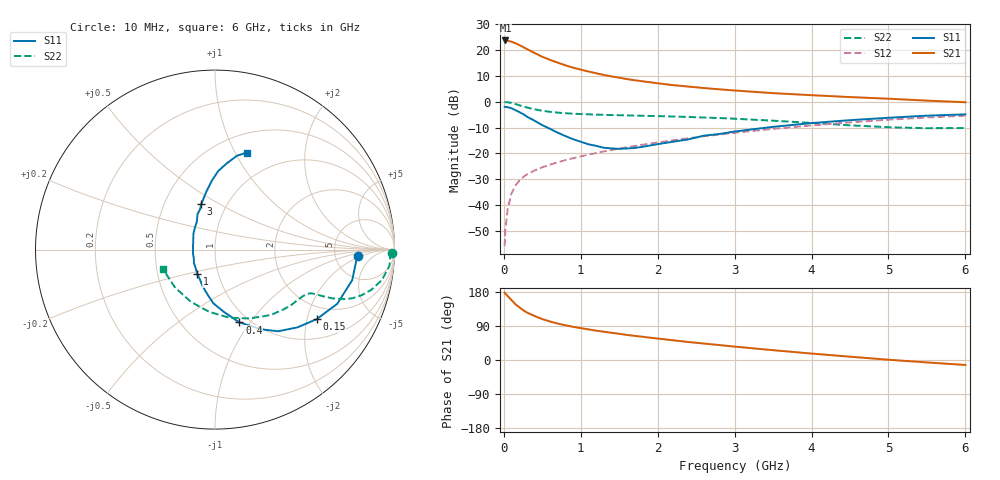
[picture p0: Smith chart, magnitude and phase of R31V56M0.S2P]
! SIEMENS Small Signal Semiconductors
! BFR181
! Si NPN RF Bipolar Junction Transistor in SOT23
! VCE = 1.5 V  IC = 6 mA
! Common Emitter S-Parameters:  May  1996
# GHz  S  MA  R  50
!  f  S11  S21  S12  S22
! GHz  MAG  ANG  MAG  ANG  MAG  ANG  MAG  ANG
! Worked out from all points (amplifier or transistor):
!   36 points, 10 MHz to 6 GHz, reference 50 ohm
!   highest |S21| = 23.7 dB at 20 MHz (marker M1)
!   |S21| within 3 dB of that: start of sweep to 279.5 MHz
!   unconditionally stable (mu >= 1): 886.1 MHz to 2.894 GHz
!   at 250 MHz: K = 0.48, MSG = 25.2 dB, |S12| = -29.2 dB
!   at 1.4 GHz: K = 1.07, MAG = 12.6 dB, |S12| = -18.7 dB
!   at 6 GHz: K = 0.87, MSG = 2.6 dB, |S12| = -5.4 dB
!   S11 on the Smith chart (normalised r, x): 10 MHz: 8.47, -1.67; 150 MHz: 1.56, -2.29; 400 MHz: 0.90, -0.89; 1 GHz: 0.79, -0.22; 3 GHz: 0.76, +0.41; 6 GHz: 0.70, +1.11
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0.01  0.7961 -2.6  15.27 177.8  0.0016 90.7  0.9874 -1.0
0.02  0.7888 -4.8  15.3 175.2  0.0033 85.3  0.9775 -2.2
0.05  0.7834 -12.5  15.13 168.7  0.0085 85.1  0.9759 -5.4
0.1  0.7452 -23.9  14.46 158.1  0.0168 78.3  0.9453 -10.3
0.15  0.6863 -34.4  13.54 147.3  0.0237 73.3  0.8999 -14.4
0.2  0.6317 -43.3  12.49 139.3  0.0297 69.5  0.8555 -17.3
0.25  0.5752 -52.3  11.43 131.7  0.0347 67.0  0.8125 -19.5
0.3  0.5131 -59.9  10.44 125.3  0.0391 65.8  0.7727 -20.9
0.4  0.4277 -71.5  8.753 116.0  0.0466 63.9  0.71 -22.5
0.5  0.3511 -81.8  7.4 107.9  0.0537 63.3  0.6675 -23.2
0.6  0.2986 -91.9  6.443 101.6  0.0605 63.6  0.6364 -23.6
0.7  0.2518 -99.8  5.692 96.2  0.0672 64.0  0.6141 -24.0
0.8  0.2159 -108.5  5.053 91.6  0.0739 64.3  0.5976 -24.2
1  0.1678 -125.7  4.168 84.1  0.0873 64.9  0.5765 -25.2
1.1  0.1499 -135.8  3.838 80.8  0.0946 65.3  0.5691 -25.9
1.6  0.1243 171.8  2.739 66.2  0.1313 65.3  0.5429 -30.4
2.2  0.1678 131.3  2.091 52.0  0.1794 63.2  0.5164 -38.3
3  0.2647 106.8  1.646 35.3  0.25 57.9  0.4679 -51.9
3.5  0.3261 98.5  1.463 25.9  0.2975 53.5  0.4291 -63.4
4.5  0.4387 87.6  1.228 8.7  0.3976 42.6  0.3488 -95.2
5.5  0.5365 76.9  1.048 -6.4  0.4943 29.5  0.3067 -137.0
6  0.5689 71.9  0.976 -13.1  0.5366 22.3  0.3092 -159.2
